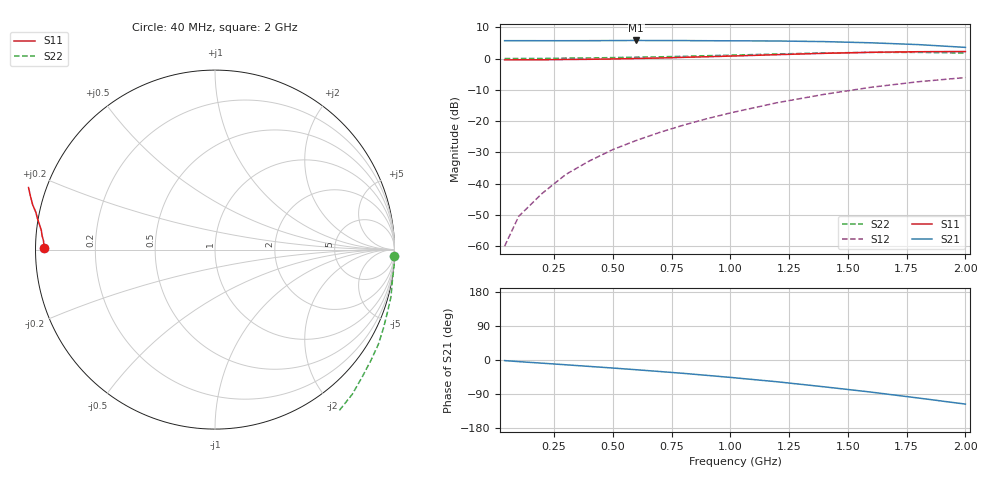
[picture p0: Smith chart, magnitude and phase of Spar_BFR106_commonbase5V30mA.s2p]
! Filename:  BFR106CB.S2P  Version:  2.0
! NXP part #: BFR106  Date: Jul 1990
! Bias condition: Vce=5V, Ic=30mA
! COMMON BASE
#  MHz  S  MA  R  50
! Freq  S11  S21  S12  S22
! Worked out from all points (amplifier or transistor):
!   16 points, 40 MHz to 2 GHz, reference 50 ohm
!   highest |S21| = 5.8 dB at 600 MHz (marker M1)
!   |S21| within 3 dB of that: start of sweep to end of sweep
!   unconditionally stable (mu >= 1): nowhere
!   at 200 MHz: K = -0.56, MSG = 24.4 dB, |S12| = -43.1 dB
!   at 800 MHz: K = -0.93, MSG = 13.5 dB, |S12| = -21.3 dB
!   at 2 GHz: K = -0.82, MSG = 4.8 dB, |S12| = -6.1 dB
40  0.952 179.5  1.932 -1.6  0.001 66.7  1 -1.9
100  0.954 178.2  1.932 -4.3  0.003 106.3  1.002 -4.8
200  0.957 177.0  1.929 -8.4  0.007 120.3  1.003 -9.7
300  0.966 175.5  1.929 -12.6  0.014 131.3  1.015 -15.0
400  0.973 173.8  1.933 -16.9  0.023 138.9  1.022 -19.8
500  0.985 172.2  1.937 -21.2  0.035 139.3  1.036 -25.1
600  1.003 170.2  1.947 -25.7  0.049 140.3  1.052 -30.1
700  1.02 168.2  1.937 -30.4  0.066 140.2  1.066 -35.5
800  1.046 166.2  1.938 -35.2  0.086 139.3  1.085 -41.0
900  1.069 164.0  1.928 -40.5  0.109 137.7  1.111 -46.5
1000  1.095 161.6  1.923 -45.9  0.135 135.2  1.133 -52.4
1200  1.154 156.2  1.909 -57.5  0.197 129.1  1.183 -64.7
1400  1.213 149.4  1.866 -70.8  0.268 121.9  1.229 -77.7
1600  1.259 141.9  1.785 -84.8  0.348 113.8  1.255 -91.3
1800  1.286 133.5  1.671 -100.3  0.426 104.3  1.256 -105.8
2000  1.295 125.9  1.509 -116.4  0.497 95.1  1.225 -120.5
